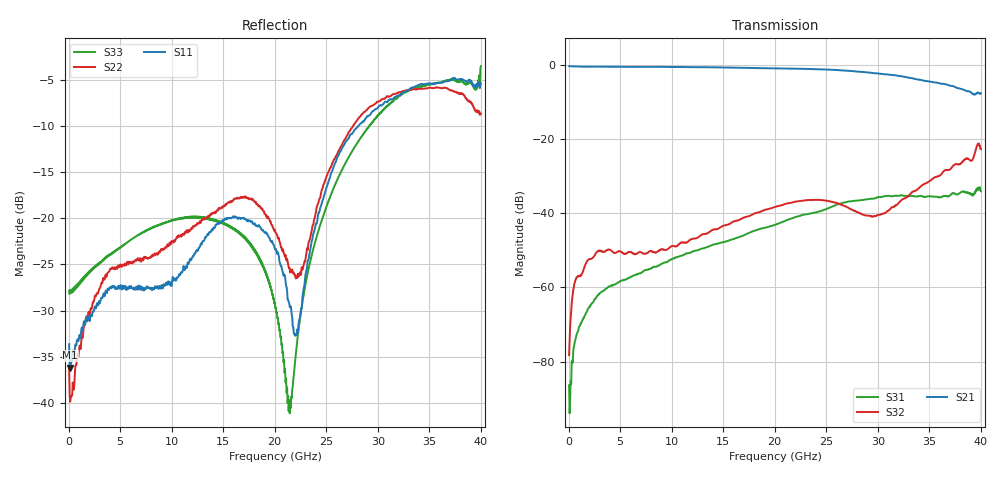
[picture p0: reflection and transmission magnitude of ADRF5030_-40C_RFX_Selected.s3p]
! Device  : ADRF5030
! Description: Silicon SPDT Switch Non-Reflective
! Frequency:  100 MHz -  20 GHz
! Ports:
!  RFC = Port 1
!  RF1 = Port 2
!  RF2 = Port 3
! VSS  =  -3.30 Volts
! VDD  =  +3.30 Volts
! EN  =  0.00 Volts
! LS  =  0.00 Volts
! V1  =  +3.30 Volts
! Data:  Data was collected using an calibrated 4 port network analyzer.
! Notes: Analog Devices supplies this data as a sample of measured data
!  for this product.  Your particular data for this product may vary.
!  Data was taken at -40 degrees C.
!  Analog Devices reserves the right to change this data at anytime.
# HZ S DB R 50
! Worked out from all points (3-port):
!   800 points, 50 MHz to 40 GHz, reference 50 ohm
!   strongest paths, dB at 50 MHz, 10.05 GHz, 20.05 GHz, 30.05 GHz, 40 GHz:
!     S21: -0.4, -0.6, -1.0, -2.4, -7.7
!     S32: -78.2, -48.8, -38.3, -40.4, -22.7
!     S31: -86.4, -52.3, -43.1, -35.6, -34.1
!   lowest |S11| = -36.2 dB at 150 MHz (marker M1), VSWR 1.03, Z = 51.6 - j0.0634 ohm
!   |S11| at or under -10 dB: start of sweep to 28.09 GHz
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5e7  -33.64 -8.6  -0.37 -0.3  -86.37 -85.6
     -0.37 -0.3  -36.15 -17.4  -78.24 36.6
     -86.37 -85.6  -78.24 36.6  -27.83 0.1
1.5e8  -36.17 -2.3  -0.38 -2.1  -90.28 -170.5
       -0.38 -2.1  -39.88 -15.1  -70.35 65.4
       -90.28 -170.5  -70.35 65.4  -27.81 -0.5
1.85e9  -30.98 -70.6  -0.51 -26.6  -65.87 90.2
        -0.51 -26.6  -30.69 -83.2  -52.70 45.1
        -65.87 90.2  -52.70 45.1  -25.90 -24.1
6.2e9  -27.61 173.6  -0.55 -89.0  -56.95 63.2
       -0.55 -89.0  -24.89 -149.5  -50.79 1.0
       -56.95 63.2  -50.79 1.0  -22.19 -85.1
1.195e10  -24.31 21.5  -0.60 -172.5  -50.40 42.8
          -0.60 -172.5  -21.03 -176.0  -46.95 -13.2
          -50.40 42.8  -46.95 -13.2  -19.94 -136.3
2.005e10  -23.40 -113.0  -0.96 64.9  -43.12 -15.9
          -0.96 64.9  -21.49 111.5  -38.27 -78.9
          -43.12 -15.9  -38.27 -78.9  -29.71 167.2
2.145e10  -29.59 -109.7  -1.03 42.7  -41.56 -34.5
          -1.03 42.7  -25.39 121.5  -37.23 -93.1
          -41.56 -34.5  -37.23 -93.1  -41.13 -126.3
2.905e10  -8.93 -96.0  -2.08 -78.5  -36.23 -164.4
          -2.08 -78.5  -8.12 114.2  -40.62 130.3
          -36.23 -164.4  -40.62 130.3  -10.21 -119.9
3.71e10  -4.97 153.3  -5.68 162.4  -35.00 97.6
         -5.68 162.4  -6.15 -13.3  -27.95 -44.9
         -35.00 97.6  -27.95 -44.9  -5.01 119.3
4e10  -5.36 19.8  -7.65 59.5  -34.06 49.4
      -7.65 59.5  -8.65 -145.0  -22.71 -169.6
      -34.06 49.4  -22.71 -169.6  -3.50 -35.4
